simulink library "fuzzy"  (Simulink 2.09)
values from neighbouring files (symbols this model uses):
  a = -1    [HdataM.m]
  alpha = 4    [VdataM.m]
  b = 1    [HdataM.m]
  ce_n = [-1 -0.5 0 0.5 1]    [HdataF.m]    (also in Mdata.m = e_n; Mdata25.m = e_n; VdataF.m = e_n; VdataF25.m = e_n)
  ceNorm = 0.033    [HdataF.m]    (also in Mdata.m = 1; Mdata25.m = 1; VdataF.m = 0.2; VdataF25.m = 0.2)
  e_n = [-1 -0.5 0 0.5 1]    [HdataF.m]    (also in Mdata.m = [-1 -0.25 0 0.25 1]; Mdata25.m = [-1 -0.5 -0.25 0 0.25 0.5 1]; VdataF.m = [-1 -0.25 0 0.25 1]; VdataF25.m = [-1 -0.5 -0.25 0 0.25 0.5 1])
  eNorm = 0.033    [HdataF.m]    (also in Mdata.m = 1; Mdata25.m = 1; VdataF.m = 0.1; VdataF25.m = 0.1)
  Fe0 = Fi+gamma*sqrt(theta0)    [VdataM.m]
  Fg = 0    [VdataM.m]
  Fi = 1000    [VdataM.m]
  gamma = 12500    [VdataM.m]
  gamma1 = 0    [VdataM.m]
  gamma3 = 0    [VdataM.m]
  LN = [1 1 0 0 0 0 0]    [Mdata25.m]    (also in VdataF25.m)
  LP = [0 0 0 0 0 1 1]    [Mdata25.m]    (also in VdataF25.m)
  m = 1000    [VdataM.m]
  N = [1 1 0 0 0]    [HdataF.m]    (also in Mdata.m; VdataF.m)
  P = [0 0 0 1 1]    [HdataF.m]    (also in Mdata.m; VdataF.m)
  Qt = 10    [HdataM.m]
  SN = [0 0 1 0 0 0 0]    [Mdata25.m]    (also in VdataF25.m)
  SP = [0 0 0 0 1 0 0]    [Mdata25.m]    (also in VdataF25.m)
  T = 2.5    [HdataF.m]    (also in Mdata.m = 0.5; Mdata25.m = 0.5; VdataC.m = 0.25; VdataF.m = 0.25)
  T0 = 50    [HdataM.m]
  Tc = 0    [HdataM.m]
  te_n = 0.1    [VdataM.m]
  te_p = 1    [VdataM.m]
  Th = 100    [HdataM.m]
  theta0 = ((1/gamma)*(alpha*v0^2-Fi))^2    (= 0.186624)    [VdataM.m]
  thetamax = pi/3    (= 1.0471975512)    [VdataM.m]
  u0 = 0    [HdataF.m]    (also in Mdata.m; Mdata25.m; VdataF.m = theta0; VdataF25.m = theta0)
  uDenorm = 0.05    [HdataF.m]    (also in Mdata.m = 1; Mdata25.m = 1; VdataF.m = 0.1; VdataF25.m = 0.1)
  uLN = -1    [Mdata25.m]    (also in VdataF25.m)
  uLP = 1    [Mdata25.m]    (also in VdataF25.m)
  uN = -1    [Mdata.m]    (also in VdataF.m)
  uP = 1    [Mdata.m]    (also in VdataF.m)
  uSN = -0.5    [Mdata25.m]    (also in VdataF25.m)
  uSP = 0.5    [Mdata25.m]    (also in VdataF25.m)
  uZ = 0    [Mdata.m]    (also in Mdata25.m; VdataF.m; VdataF25.m)
  v0 = 40    [VdataM.m]
  Z = [0 0 1 0 0]    [HdataF.m]    (also in Mdata.m; Mdata25.m = [0 0 0 1 0 0 0]; VdataF.m; VdataF25.m = [0 0 0 1 0 0 0])
undefined symbols (not defined in the file or in its folder): i1, i2, nb, nm, pb, pm, x, ze, zi
libraries: fuzzy x6
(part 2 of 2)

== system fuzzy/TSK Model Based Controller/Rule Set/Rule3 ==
  in_1 : Inport  Port=1  PortWidth=-1  SampleTime=-1
  in_2 : Inport  Port=2  PortWidth=-1  SampleTime=-1
  PB : Lookup  InputValues=x  OutputValues=pb
  Product1 : Product  Inputs=2
  Z2 : Lookup  InputValues=i2  OutputValues=zi
  out_1 : Outport  Port=1  InitialOutput=0
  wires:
  in_2/1 -> Z2/1
  Product1/1 -> out_1/1
  in_1/1 -> PB/1
  PB/1 -> Product1/1
  Z2/1 -> Product1/2

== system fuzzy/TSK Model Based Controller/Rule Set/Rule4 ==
  in_1 : Inport  Port=1  PortWidth=-1  SampleTime=-1
  in_2 : Inport  Port=2  PortWidth=-1  SampleTime=-1
  NM1 : Lookup  InputValues=i1  OutputValues=nm
  PM : Lookup  InputValues=x  OutputValues=pm
  Product : Product  Inputs=2
  out_1 : Outport  Port=1  InitialOutput=0
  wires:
  in_2/1 -> NM1/1
  Product/1 -> out_1/1
  in_1/1 -> PM/1
  PM/1 -> Product/1
  NM1/1 -> Product/2

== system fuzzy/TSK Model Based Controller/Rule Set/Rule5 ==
  in_1 : Inport  Port=1  PortWidth=-1  SampleTime=-1
  in_2 : Inport  Port=2  PortWidth=-1  SampleTime=-1
  NM2 : Lookup  InputValues=i2  OutputValues=nm
  PB : Lookup  InputValues=x  OutputValues=pb
  Product2 : Product  Inputs=2
  out_1 : Outport  Port=1  InitialOutput=0
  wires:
  in_2/1 -> NM2/1
  Product2/1 -> out_1/1
  in_1/1 -> PB/1
  PB/1 -> Product2/1
  NM2/1 -> Product2/2

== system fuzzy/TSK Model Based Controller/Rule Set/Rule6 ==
  in_1 : Inport  Port=1  PortWidth=-1  SampleTime=-1
  in_2 : Inport  Port=2  PortWidth=-1  SampleTime=-1
  NB1 : Lookup  InputValues=i1  OutputValues=nb
  PM : Lookup  InputValues=x  OutputValues=pm
  Product : Product  Inputs=2
  out_1 : Outport  Port=1  InitialOutput=0
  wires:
  in_2/1 -> NB1/1
  Product/1 -> out_1/1
  in_1/1 -> PM/1
  PM/1 -> Product/1
  NB1/1 -> Product/2

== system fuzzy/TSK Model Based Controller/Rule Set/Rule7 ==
  in_1 : Inport  Port=1  PortWidth=-1  SampleTime=-1
  in_2 : Inport  Port=2  PortWidth=-1  SampleTime=-1
  NB2 : Lookup  InputValues=i2  OutputValues=nb
  PB : Lookup  InputValues=x  OutputValues=pb
  Product2 : Product  Inputs=2
  out_1 : Outport  Port=1  InitialOutput=0
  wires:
  in_2/1 -> NB2/1
  Product2/1 -> out_1/1
  in_1/1 -> PB/1
  PB/1 -> Product2/1
  NB2/1 -> Product2/2

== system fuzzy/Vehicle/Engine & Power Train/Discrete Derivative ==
  e : Inport  Port=1  PortWidth=-1  SampleTime=-1
  Sum1 : Sum  Inputs=+-
  Unit Delay : UnitDelay  X0=0  SampleTime=T
  ce : Outport  Port=1  InitialOutput=0
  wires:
  e/1 -> Unit Delay/1, Sum1/1
  Sum1/1 -> ce/1
  Unit Delay/1 -> Sum1/2
